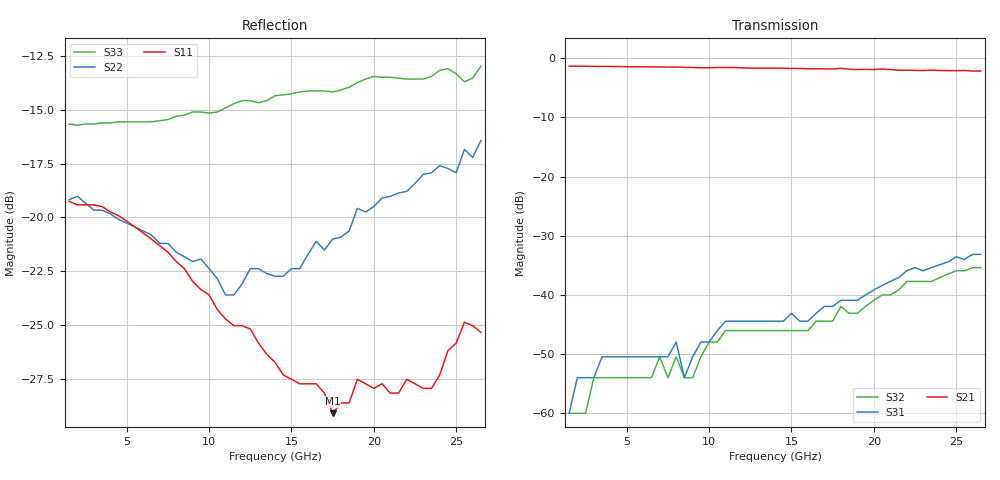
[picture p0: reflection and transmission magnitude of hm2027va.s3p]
! HMMC-2027
! S-PARAMETERS at  Vsel high = 0V; Vsel low = -10V.  LAST UPDATED  02-06-97
# GHZ  S  MA  R  50
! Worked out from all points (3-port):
!   51 points, 1.5 GHz to 26.5 GHz, reference 50 ohm
!   strongest paths, dB at 1.5 GHz, 7.5 GHz, 14 GHz, 20.5 GHz, 26.5 GHz:
!     S21: -1.4, -1.5, -1.7, -1.8, -2.2
!     S31: -60.0, -50.5, -44.4, -38.4, -33.2
!     S32: -60.0, -54.0, -46.0, -40.0, -35.4
!   lowest |S11| = -29.1 dB at 17.5 GHz (marker M1), VSWR 1.07, Z = 46.6 + j4e-16 ohm
!   |S11| at or under -10 dB: start of sweep to end of sweep
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1.5  0.109 -14.0  0.856 -16.0  0.001 85.0
     0.856 -16.0  0.11 -22.0  0.001 69.0
     0.001 85.0  0.001 69.0  0.165 162.0
2  0.107 -18.0  0.856 -19.0  0.002 70.0
   0.856 -19.0  0.112 -28.0  0.001 51.0
   0.002 70.0  0.001 51.0  0.164 158.0
3.5  0.106 -24.0  0.852 -23.0  0.003 70.0
     0.852 -23.0  0.104 -37.0  0.002 47.0
     0.003 70.0  0.002 47.0  0.166 154.0
7.5  0.083 -53.0  0.841 -48.0  0.003 53.0
     0.841 -48.0  0.087 -84.0  0.002 5.0
     0.003 53.0  0.002 5.0  0.169 129.0
8  0.079 -57.0  0.842 -51.0  0.004 54.0
   0.842 -51.0  0.083 -90.0  0.003 3.0
   0.004 54.0  0.003 3.0  0.172 126.0
8.5  0.076 -62.0  0.836 -55.0  0.002 67.0
     0.836 -55.0  0.081 -99.0  0.002 13.0
     0.002 67.0  0.002 13.0  0.173 123.0
11  0.058 -78.0  0.834 -72.0  0.006 59.0
    0.834 -72.0  0.066 -139.0  0.005 -12.0
    0.006 59.0  0.005 -12.0  0.18 108.0
14  0.046 -123.0  0.824 -88.0  0.006 45.0
    0.824 -88.0  0.073 171.0  0.005 -43.0
    0.006 45.0  0.005 -43.0  0.192 98.0
17.5  0.035 180.0  0.81 -113.0  0.008 43.0
      0.81 -113.0  0.089 113.0  0.006 -70.0
      0.008 43.0  0.006 -70.0  0.196 81.0
26.5  0.054 -164.0  0.779 -178.0  0.022 3.0
      0.779 -178.0  0.151 -20.0  0.017 -176.0
      0.022 3.0  0.017 -176.0  0.225 44.0
